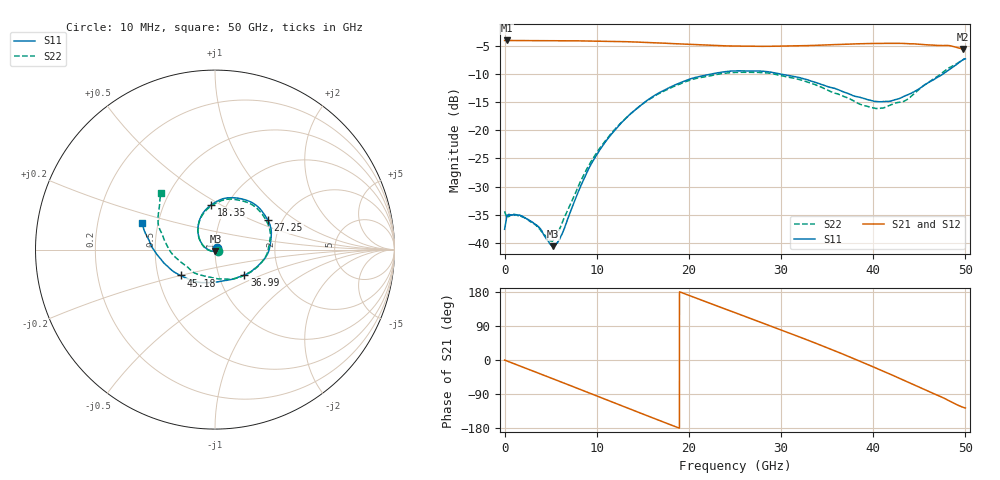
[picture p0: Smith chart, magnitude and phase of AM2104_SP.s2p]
!Keysight Technologies,N5245B,MY58422270,A.16.20.02
!Date: Thursday, March 12, 2026 18:27:18
!Correction: S11(C  2-Port  )
!S21(C  2-Port  )
!S12(C  2-Port  )
!S22(C  2-Port  )
!S2P File: Measurements: S11, S21, S12, S22:
# Hz S  dB  R 50
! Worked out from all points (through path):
!   6401 points, 10 MHz to 50 GHz, reference 50 ohm
!   highest |S21| = -4.01 dB at 283.4 MHz (marker M1); lowest = -5.5 dB at 49.76 GHz (marker M2)
!   group delay of S21, straight-line fit = 26.6 ps
!   lowest |S11| = -40.6 dB at 5.282 GHz (marker M3), VSWR 1.02, Z = 50.2 - j0.911 ohm
!   |S11| at or under -10 dB: start of sweep to 22.36 GHz; 29.97 GHz to 47.54 GHz (17.57 GHz wide, 45.3 % of centre)
!   |S22| runs from -39.7 to -7.2 dB; largest |S21 - S12| = 0.0074
!   S11 on the Smith chart (normalised r, x): 10 MHz: 1.02, +0.02; 18.35 GHz: 0.85, +0.45; 27.25 GHz: 1.69, +0.62; 36.99 GHz: 1.32, -0.39; 45.18 GHz: 0.65, -0.20; 50 GHz: 0.41, +0.15
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1e7  -37.61 47.8  -4.01 -0.3  -4.02 -0.7  -34.39 -17.5
2.833828e8  -35.14 0.0  -4.01 -2.7  -4.02 -2.7  -35.52 -0.8
2.829748e9  -36.13 -16.3  -4.04 -26.8  -4.04 -26.8  -36.30 -21.3
5.282383e9  -40.61 -76.7  -4.06 -49.9  -4.05 -49.9  -39.57 -91.4
6.149397e9  -38.73 -119.7  -4.06 -58.1  -4.06 -58.1  -36.83 -128.4
8.34427e9  -29.64 -175.7  -4.08 -78.9  -4.08 -78.9  -28.79 -175.6
9.945512e9  -24.48 166.2  -4.12 -94.2  -4.11 -94.2  -24.13 166.7
1.178889e10  -20.31 149.1  -4.17 -111.8  -4.17 -111.8  -20.15 148.8
1.667854e10  -13.40 108.3  -4.45 -158.3  -4.45 -158.3  -13.52 107.9
1.835008e10  -12.03 94.9  -4.58 -174.1  -4.58 -174.1  -12.21 94.7
2.15057e10  -10.29 70.9  -4.80 156.8  -4.80 156.8  -10.54 70.7
2.5005e10  -9.44 45.2  -5.00 125.0  -4.99 125.0  -9.69 44.6
2.724674e10  -9.43 28.9  -5.05 104.6  -5.05 104.6  -9.70 27.8
3.025395e10  -10.09 8.2  -5.01 77.2  -5.00 77.3  -10.35 5.3
3.333927e10  -11.28 -13.2  -4.91 48.3  -4.89 48.3  -11.67 -19.3
3.698698e10  -13.30 -40.9  -4.69 12.8  -4.68 12.7  -14.09 -54.0
3.932245e10  -14.50 -62.5  -4.57 -11.1  -4.56 -11.1  -15.72 -84.3
4.167354e10  -14.86 -91.3  -4.53 -35.7  -4.52 -35.7  -15.63 -122.2
4.518065e10  -12.39 -143.1  -4.71 -73.9  -4.71 -73.9  -12.40 -174.1
4.787542e10  -9.63 -176.8  -4.91 -103.1  -4.89 -103.0  -9.27 156.6
4.975786e10  -7.40 161.2  -5.53 -125.0  -5.53 -125.0  -7.43 135.6
5e10  -7.28 159.9  -5.52 -126.6  -5.64 -126.4  -7.23 133.5
